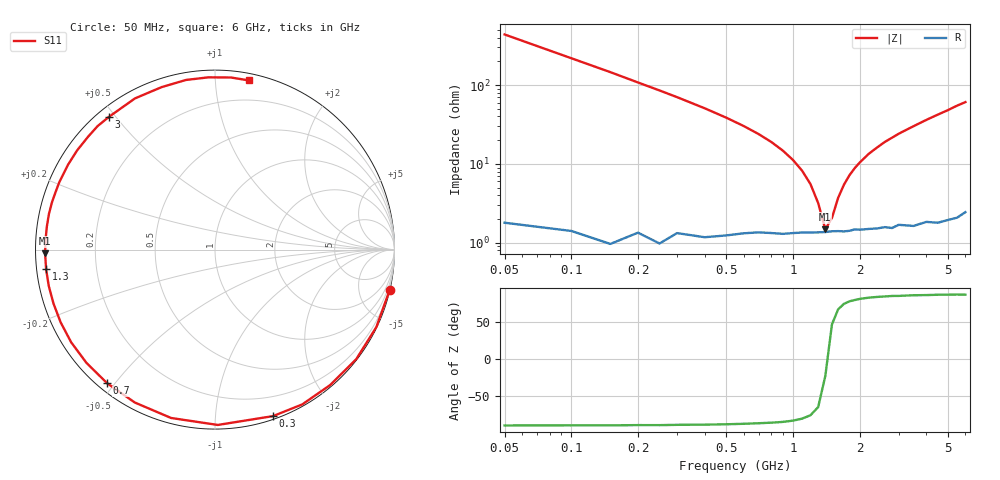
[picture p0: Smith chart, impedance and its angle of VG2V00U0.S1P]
! Infineon Technologies  Discrete & RF Semiconductors
! BB 831
! Si Tuning Diode in SOD323
! VR = 2 V
! S-Parameters:  July  1999
# GHz  S  MA  R  50
!  f  S11
! GHz  MAG  ANG
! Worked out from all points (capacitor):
!   34 points, 50 MHz to 6 GHz, reference 50 ohm
!   read as one part to ground: C = 7.23 pF near 50 MHz
!   lowest |Z| = 1.48 ohm at 1.4 GHz (marker M1)
!   series resonance near 1.427 GHz, so ESL is about 1.7 nH
!   S11 on the Smith chart (normalised r, x): 50 MHz: 0.04, -8.78; 300 MHz: 0.03, -1.41; 700 MHz: 0.03, -0.48; 1.3 GHz: 0.03, -0.06; 3 GHz: 0.03, +0.48; 6 GHz: 0.05, +1.22
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0.05  0.9991 -13.0
0.1  0.9972 -25.7
0.15  0.996 -37.8
0.2  0.9906 -49.7
0.25  0.9901 -60.6
0.3  0.9823 -70.8
0.4  0.9771 -89.1
0.5  0.9694 -104.6
0.6  0.9621 -117.7
0.7  0.9568 -128.9
0.8  0.9546 -138.6
0.9  0.9534 -147.2
1  0.9507 -154.8
1.1  0.9487 -161.6
1.3  0.9473 -173.4
1.4  0.9468 -178.7
1.6  0.9456 172.1
1.8  0.9459 163.9
2  0.9453 156.7
2.4  0.9464 144.2
2.6  0.9463 138.4
3  0.9466 128.5
3.5  0.9531 117.9
4  0.9528 108.2
4.5  0.9589 99.7
5  0.9604 92.2
5.5  0.9629 84.7
6  0.9613 78.8
